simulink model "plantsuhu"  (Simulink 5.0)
settings: Solver=ode45  StartTime=0.0  StopTime=500  RelTol=1e-3

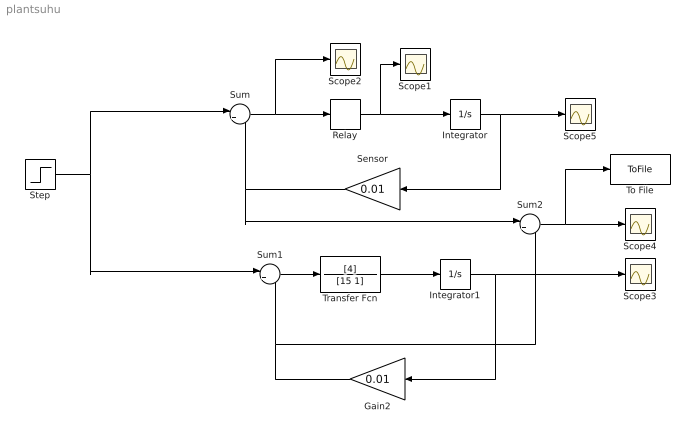
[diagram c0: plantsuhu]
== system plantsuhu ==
  Gain2 : Gain  Orientation=left  Gain=0.01
  Integrator : Integrator  InitialCondition=25
  Integrator1 : Integrator  InitialCondition=25
  Relay : Relay  OnSwitchValue=.02  OffSwitchValue=-.02  OnOutputValue=0.366  OffOutputValue=-0.057
  Scope{1..5} (5 alike) : Scope
  Sensor : Gain  Orientation=left  Gain=0.01
  Step : Step  Time=0  After=0.5  SampleTime=0
  Sum : Sum  Inputs=|+-
  Sum1 : Sum  Inputs=|+-
  Sum2 : Sum  Inputs=|+-
  To File : ToFile  Filename=data.mat  MatrixName=data
  Transfer Fcn : TransferFcn  Numerator=[4]  Denominator=[15 1]
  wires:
  Sum/1 -> Scope2/1, Relay/1
  Relay/1 -> Integrator/1, Scope1/1
  Integrator/1 -> Sensor/1, Scope5/1
  Integrator1/1 -> Gain2/1, Scope3/1
  Transfer Fcn/1 -> Integrator1/1
  Sum1/1 -> Transfer Fcn/1
  Gain2/1 -> Sum1/2, Sum2/2
  Sum2/1 -> Scope4/1, To File/1
  Step/1 -> Sum/1, Sum1/1
  Sensor/1 -> Sum/2, Sum2/1
